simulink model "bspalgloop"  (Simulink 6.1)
settings: Solver=ode45  StartTime=0.0  StopTime=10.0  FixedStep=0.0001  RelTol=1e-3
libraries: simulink x1

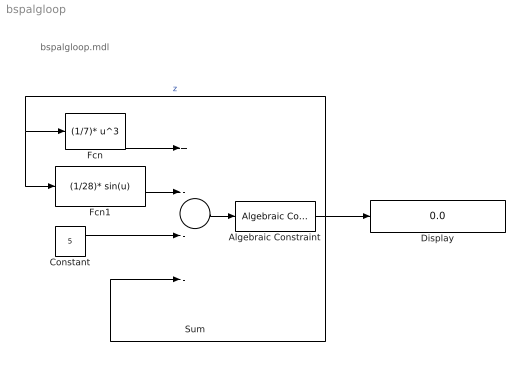
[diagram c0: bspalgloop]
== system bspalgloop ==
  note: bspalgloop.mdl
  Algebraic Constraint : simulink/Math Operations/Algebraic Constraint  z0=0
  Constant : Constant  Value=5
  Display : Display
  Fcn : Fcn  Expr=(1/7)* u^3
  Fcn1 : Fcn  Expr=(1/28)* sin(u)
  Sum : Sum  Inputs=+---
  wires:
  Fcn/1 -> Sum/1
  Fcn1/1 -> Sum/2
  Constant/1 -> Sum/3
  Sum/1 -> Algebraic Constraint/1
  Algebraic Constraint/1 -> Sum/4, Display/1, Fcn/1, Fcn1/1  "z"
